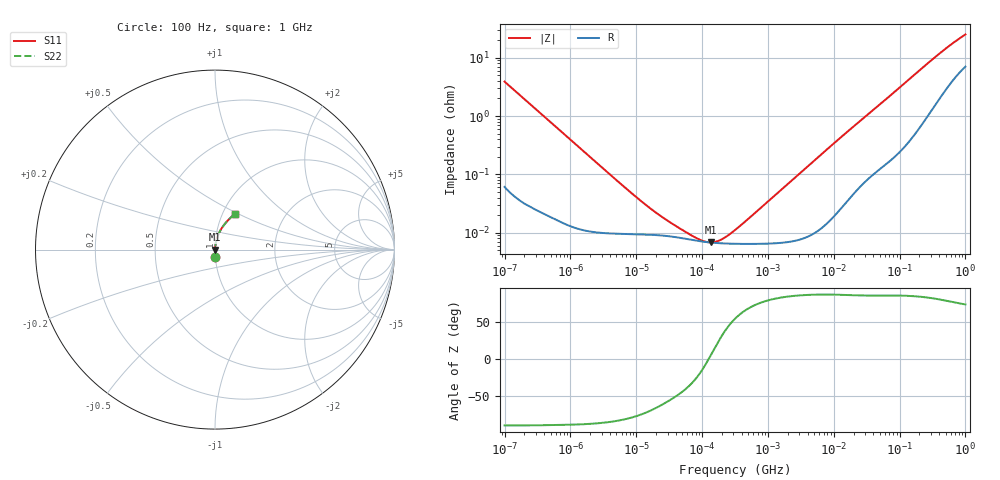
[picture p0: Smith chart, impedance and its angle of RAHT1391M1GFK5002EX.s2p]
! RAHT1391M1GFK5002EX  S-PARAMETER MODEL  (AEC-Q200 qualified)
! Model Generated by ELNA Corporation (http://www.ty-top.com)
! Version 1.0
! ELNA Control No. 201216
! Copyright (c) 2020 ELNA CO.,LTD. All Rights Reserved.
! Products Name : CONDUCTIVE POLYMER HYBRID ALUMINUM ELECTROLYTIC CAPACITORS
! Characteristics :
!  Capacitance  :  390uF  ,  Rated voltage  :  35V
!  Operating Temp. Range  :  -55 to +105 degC  ,  Endurance  :  10000hr at 105 degC
!  Dimension D  :  10mm  ,  Dimension L  :  12.5mm
! Frequency Range : 100Hz - 1GHz
! External Node Assignments :
!  1  o---| |---o  2
# MHz S RI R 50
!Freq[MHz].  S11 Real  S11 Imag  S21 Real  S21 Imag  S12 Real  S12 Imag  S22 Real  S22 Imag
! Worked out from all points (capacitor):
!   401 points, 100 Hz to 1 GHz, reference 50 ohm
!   read as one part in series: C = 410 uF near 108 Hz
!   lowest |Z| = 6.85 mohm at 135.7 kHz (marker M1)
!   series resonance near 125.5 kHz, so ESL is about 3.9 nH
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0.0001  0.00211 -0.0387  0.9979 0.0387  0.9979 0.0387  0.00211 -0.0387
0.000113  0.00171 -0.0343  0.9983 0.0343  0.9983 0.0343  0.00171 -0.0343
0.000285  0.000441 -0.0137  0.9996 0.0137  0.9996 0.0137  0.000441 -0.0137
0.001488  0.00012 -0.00265  0.9999 0.00265  0.9999 0.00265  0.00012 -0.00265
0.00876  9.51e-05 -0.000454  0.9999 0.000454  0.9999 0.000454  9.51e-05 -0.000454
0.014207  9.34e-05 -0.000281  0.9999 0.000281  0.9999 0.000281  9.34e-05 -0.000281
0.022131  9.08e-05 -0.000182  0.9999 0.000182  0.9999 0.000182  9.08e-05 -0.000182
0.037368  8.51e-05 -0.000108  0.9999 0.000108  0.9999 0.000108  8.51e-05 -0.000108
0.05821  7.85e-05 -6.37e-05  0.9999 6.37e-05  0.9999 6.37e-05  7.85e-05 -6.37e-05
0.06569  7.66e-05 -5.31e-05  0.9999 5.31e-05  0.9999 5.31e-05  7.66e-05 -5.31e-05
0.135675  6.82e-05 6.46e-06  0.9999 -6.46e-06  0.9999 -6.46e-06  6.82e-05 6.46e-06
0.258523  6.52e-05 6.69e-05  0.9999 -6.69e-05  0.9999 -6.69e-05  6.52e-05 6.69e-05
0.291743  6.5e-05 8.07e-05  0.9999 -8.07e-05  0.9999 -8.07e-05  6.5e-05 8.07e-05
0.316228  6.49e-05 9.05e-05  0.9999 -9.05e-05  0.9999 -9.05e-05  6.49e-05 9.05e-05
0.60256  6.46e-05 0.000197  0.9999 -0.000197  0.9999 -0.000197  6.46e-05 0.000197
4.704354  9.62e-05 0.00161  0.9999 -0.00161  0.9999 -0.00161  9.62e-05 0.00161
15.13561  0.000348 0.00506  0.9997 -0.00506  0.9997 -0.00506  0.000348 0.00506
69.9842  0.00213 0.0216  0.9979 -0.0216  0.9979 -0.0216  0.00213 0.0216
176.8072  0.00791 0.0527  0.9921 -0.0527  0.9921 -0.0527  0.00791 0.0527
395.8221  0.0309 0.1084  0.9691 -0.1084  0.9691 -0.1084  0.0309 0.1084
668.3439  0.068 0.1586  0.932 -0.1586  0.932 -0.1586  0.068 0.1586
1000  0.1102 0.1993  0.8898 -0.1993  0.8898 -0.1993  0.1102 0.1993
